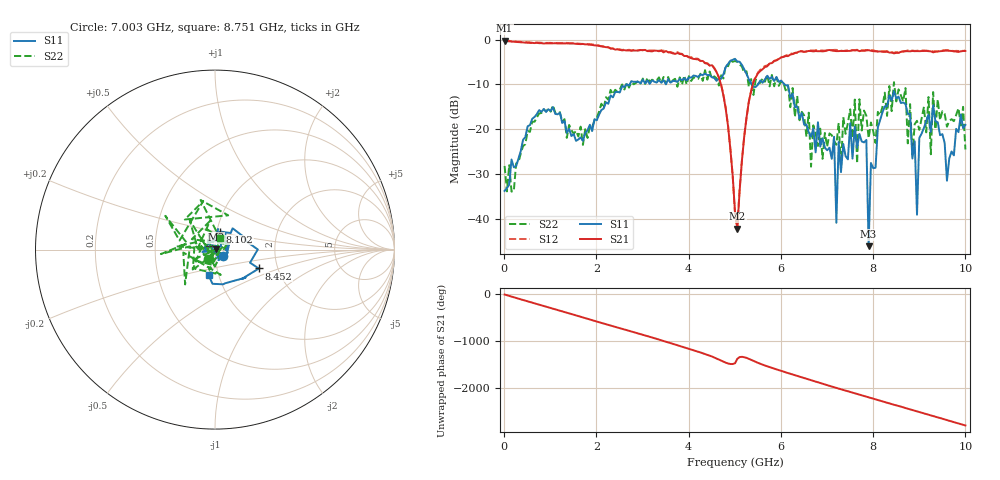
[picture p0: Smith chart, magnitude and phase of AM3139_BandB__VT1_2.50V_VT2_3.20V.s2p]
! Date/Time: Tue, Nov 13, 2018 5:00 PM
! Network Analyzer: Agilent Technologies E8364B Rev: A.07.50.67
! Sweep from 0.010 to 10.000 GHz, 201 Points, Sweep Type: LIN
! Power Supply: 2.501 V, 0.000 A
# Hz S DB R 50
!freq MagS11 AngS11 MagS21 AngS21 MagS12 AngS12 MagS22 AngS22
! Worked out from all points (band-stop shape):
!   201 points, 10 MHz to 10 GHz, reference 50 ohm
!   highest |S21| = -0.22 dB at 10 MHz (marker M1); lowest = -42.2 dB at 5.055 GHz (marker M2)
!   |S21| within 3 dB of the highest: start of sweep to 3.806 GHz; 6.259 GHz to end of sweep
!   lowest |S11| = -46.1 dB at 7.902 GHz (marker M3), VSWR 1.01, Z = 50.5 + j0.183 ohm
!   |S11| at or under -10 dB: start of sweep to 2.651 GHz; 5.371 GHz to 5.507 GHz (135.5 MHz wide, 2.49 % of centre); 6.082 GHz to end of sweep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
!   |S22| runs from -33.9 to -4.6 dB; largest |S21 - S12| = 0.031
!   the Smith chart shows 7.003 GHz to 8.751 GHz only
!   S11 on the Smith chart (normalised r, x): 7.003 GHz: 1.09, -0.08; 8.102 GHz: 1.04, +0.21; 8.452 GHz: 1.60, -0.36; 8.751 GHz: 0.89, -0.26
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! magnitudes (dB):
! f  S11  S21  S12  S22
! 10 MHz  -33.8  -0.2  -0.2  -28.2
! 1.708 GHz  -22.6  -1.0  -1.0  -23.5
! 3.357 GHz  -9.1  -2.6  -2.5  -8.4
! 4.605 GHz  -9.2  -7.3  -7.2  -8.6
! 5.005 GHz  -4.3  -38.4  -38.9  -4.8
! 5.055 GHz  -4.9  -42.2  -41.9  -5.0
! 5.405 GHz  -10.6  -9.5  -9.3  -12.4
! 6.703 GHz  -19.9  -2.6  -2.4  -19.1
! 7.003 GHz  -24.7  -2.4  -2.5  -23.9
! 7.153 GHz  -21.7  -2.5  -2.3  -22.5
! 7.203 GHz  -40.9  -2.6  -2.3  -23.5
! 7.253 GHz  -22.9  -2.6  -2.4  -18.6
! 7.852 GHz  -22.4  -2.4  -2.3  -17.0
! 7.902 GHz  -46.1  -2.4  -2.3  -22.0
! 8.102 GHz  -19.6  -2.7  -2.6  -16.1
! 8.352 GHz  -12.4  -2.9  -2.9  -10.4
! 8.452 GHz  -11.5  -3.1  -3.0  -9.5
! 8.751 GHz  -16.6  -2.6  -2.4  -23.2
! 8.951 GHz  -39.1  -2.6  -2.5  -18.1
! 9.301 GHz  -14.6  -2.9  -2.7  -11.7
! 9.6 GHz  -31.5  -2.5  -2.4  -19.4
! 10 GHz  -19.0  -2.5  -2.5  -24.5
